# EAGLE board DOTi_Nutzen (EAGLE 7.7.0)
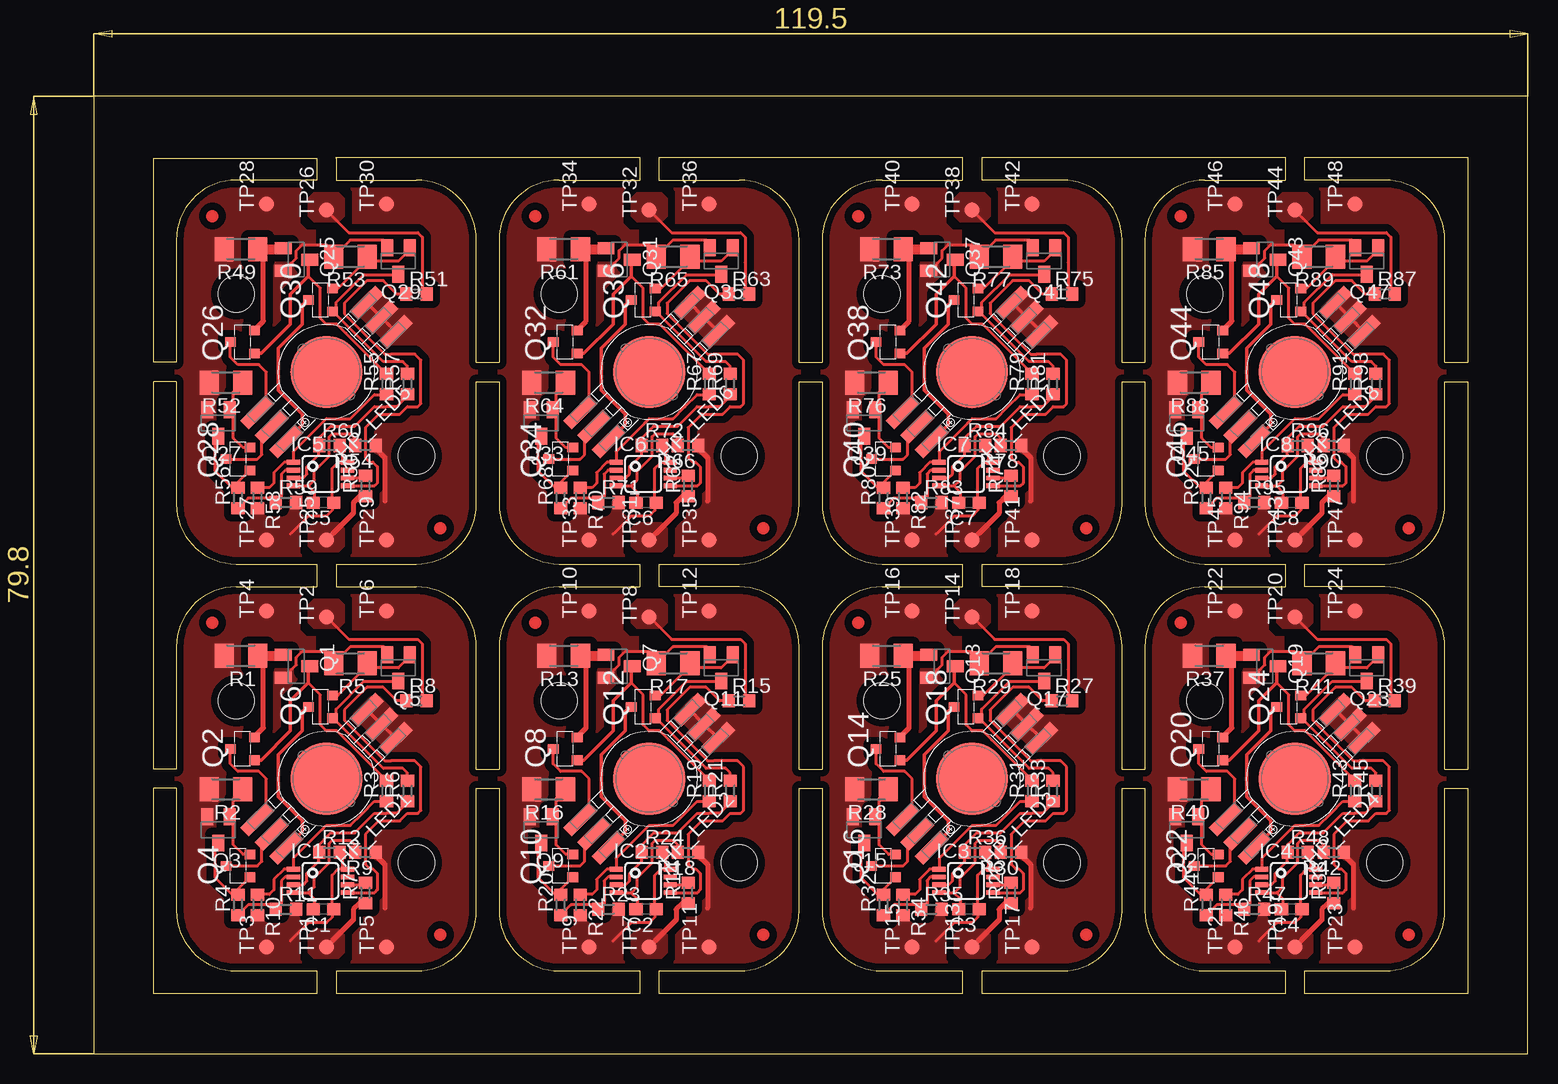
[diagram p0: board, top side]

Size 124.8 x 85.3 mm. Coordinates in mm from the lower left corner, seen from the top.
Outline: 171 segments
Copper layers (1*16): Top 0.035mm / dielectric 1.5mm / Bottom 0.035mm
Design rules "default *": minimum track width 10mil, minimum drill 24mil, track to track 8mil, track to pad 8mil, pad to pad 8mil, via to via 8mil, smd to smd 8mil, copper to edge 20mil, drill to drill 8mil, minimum pad ring 10mil, minimum via ring 8mil, stop-mask expansion 4mil, vias tented up to drill 0mil, thermal gap 10mil
Holes 3 mm at 32.2,15.9 17.2,29.4 59.1,15.9 44.1,29.4 86,15.9 71,29.4 112.9,15.9 97.9,29.4 32.2,49.8 17.2,63.3 59.1,49.8 44.1,63.3 86,49.8 71,63.3 112.9,49.8 97.9,63.3

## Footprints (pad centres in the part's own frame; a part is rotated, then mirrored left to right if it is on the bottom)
C0603 = smd 1.1 x 1: 1 -0.85,0; 2 0.85,0
HP_RGB_LED = smd 3 x 1: 1 -6.45,1.7; 2 -6.45,0; 3 -6.45,-1.7; 4 6.45,-1.7; 5 6.45,0; 6 6.45,1.7 | smd 6 x 6: P$1 0,0
MSOP8 = smd 1.1 x 0.4: 1 -2.25,0.975; 2 -2.25,0.325; 3 -2.25,-0.325; 4 -2.25,-0.975; 5 2.25,-0.975; 6 2.25,-0.325; 7 2.25,0.325; 8 2.25,0.975
SOT23-BEC = smd 1 x 1.4: B -0.95,-1.1; C 0,1.1; E 0.95,-1.1
MICRO3 = smd 0.8 x 0.9: 1 -0.95,-1; 2 0.95,-1; 3 0,1
M1206 = smd 1.6 x 2: 1 -1.4,0; 2 1.4,0
R0603 = smd 1 x 1.1: 1 -0.85,0; 2 0.85,0
B1,27 = smd 1.27 x 1.27: TP 0,0

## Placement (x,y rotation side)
C1  [C0603]  24.45,12.03 180 top
C2  [C0603]  51.35,12.03 180 top
C3  [C0603]  78.25,12.03 180 top
C4  [C0603]  105.15,12.03 180 top
C5  [C0603]  24.45,45.92 180 top
C6  [C0603]  51.35,45.92 180 top
C7  [C0603]  78.25,45.92 180 top
C8  [C0603]  105.15,45.92 180 top
HP_LED1  55-2013  [HP_RGB_LED]  24.7,22.9 225 top
HP_LED2  55-2013  [HP_RGB_LED]  51.6,22.9 225 top
HP_LED3  55-2013  [HP_RGB_LED]  78.5,22.9 225 top
HP_LED4  55-2013  [HP_RGB_LED]  105.4,22.9 225 top
HP_LED5  55-2013  [HP_RGB_LED]  24.7,56.8 225 top
HP_LED6  55-2013  [HP_RGB_LED]  51.6,56.8 225 top
HP_LED7  55-2013  [HP_RGB_LED]  78.5,56.8 225 top
HP_LED8  55-2013  [HP_RGB_LED]  105.4,56.8 225 top
IC1  [MSOP8]  24.2,14.4 0 top
IC2  [MSOP8]  51.1,14.4 0 top
IC3  [MSOP8]  78,14.4 0 top
IC4  [MSOP8]  104.9,14.4 0 top
IC5  [MSOP8]  24.2,48.3 0 top
IC6  [MSOP8]  51.1,48.3 0 top
IC7  [MSOP8]  78,48.3 0 top
IC8  [MSOP8]  104.9,48.3 0 top
Q1  BC857  [SOT23-BEC]  22.2,32.27 270 top
Q2  IRLML5203  [MICRO3]  17.7,25.4 90 top
Q3  BC857  [SOT23-BEC]  15.7,18.65 180 top
Q4  IRLML5203  [MICRO3]  17.32,15.65 90 top
Q5  BC857  [SOT23-BEC]  30.7,32.15 180 top
Q6  IRLML5203  [MICRO3]  24.2,28.9 90 top
Q7  BC857  [SOT23-BEC]  49.1,32.27 270 top
Q8  IRLML5203  [MICRO3]  44.6,25.4 90 top
Q9  BC857  [SOT23-BEC]  42.6,18.65 180 top
Q10  IRLML5203  [MICRO3]  44.22,15.65 90 top
Q11  BC857  [SOT23-BEC]  57.6,32.15 180 top
Q12  IRLML5203  [MICRO3]  51.1,28.9 90 top
Q13  BC857  [SOT23-BEC]  76,32.27 270 top
Q14  IRLML5203  [MICRO3]  71.5,25.4 90 top
Q15  BC857  [SOT23-BEC]  69.5,18.65 180 top
Q16  IRLML5203  [MICRO3]  71.12,15.65 90 top
Q17  BC857  [SOT23-BEC]  84.5,32.15 180 top
Q18  IRLML5203  [MICRO3]  78,28.9 90 top
Q19  BC857  [SOT23-BEC]  102.9,32.27 270 top
Q20  IRLML5203  [MICRO3]  98.4,25.4 90 top
Q21  BC857  [SOT23-BEC]  96.4,18.65 180 top
Q22  IRLML5203  [MICRO3]  98.02,15.65 90 top
Q23  BC857  [SOT23-BEC]  111.4,32.15 180 top
Q24  IRLML5203  [MICRO3]  104.9,28.9 90 top
Q25  BC857  [SOT23-BEC]  22.2,66.17 270 top
Q26  IRLML5203  [MICRO3]  17.7,59.3 90 top
Q27  BC857  [SOT23-BEC]  15.7,52.55 180 top
Q28  IRLML5203  [MICRO3]  17.32,49.55 90 top
Q29  BC857  [SOT23-BEC]  30.7,66.05 180 top
Q30  IRLML5203  [MICRO3]  24.2,62.8 90 top
Q31  BC857  [SOT23-BEC]  49.1,66.17 270 top
Q32  IRLML5203  [MICRO3]  44.6,59.3 90 top
Q33  BC857  [SOT23-BEC]  42.6,52.55 180 top
Q34  IRLML5203  [MICRO3]  44.22,49.55 90 top
Q35  BC857  [SOT23-BEC]  57.6,66.05 180 top
Q36  IRLML5203  [MICRO3]  51.1,62.8 90 top
Q37  BC857  [SOT23-BEC]  76,66.17 270 top
Q38  IRLML5203  [MICRO3]  71.5,59.3 90 top
Q39  BC857  [SOT23-BEC]  69.5,52.55 180 top
Q40  IRLML5203  [MICRO3]  71.12,49.55 90 top
Q41  BC857  [SOT23-BEC]  84.5,66.05 180 top
Q42  IRLML5203  [MICRO3]  78,62.8 90 top
Q43  BC857  [SOT23-BEC]  102.9,66.17 270 top
Q44  IRLML5203  [MICRO3]  98.4,59.3 90 top
Q45  BC857  [SOT23-BEC]  96.4,52.55 180 top
Q46  IRLML5203  [MICRO3]  98.02,49.55 90 top
Q47  BC857  [SOT23-BEC]  111.4,66.05 180 top
Q48  IRLML5203  [MICRO3]  104.9,62.8 90 top
R1  1R8  [M1206]  17.57,33.15 180 top
R2  1R8  [M1206]  16.32,22.02 180 top
R3  4k7  [R0603]  29.7,21.9 90 top
R4  4k7  [R0603]  17.32,12.4 90 top
R5  1R8  [M1206]  26.7,32.52 180 top
R6  4k7  [R0603]  31.45,21.9 90 top
R7  100  [R0603]  27.95,13.4 90 top
R8  100  [R0603]  32.2,29.4 0 top
R9  10  [R0603]  27.95,16.77 180 top
R10  390  [R0603]  18.95,12.4 270 top
R11  390  [R0603]  21.32,12.03 0 top
R12  390  [R0603]  24.95,16.77 0 top
R13  1R8  [M1206]  44.47,33.15 180 top
R14  100  [R0603]  54.85,13.4 90 top
R15  100  [R0603]  59.1,29.4 0 top
R16  1R8  [M1206]  43.22,22.02 180 top
R17  1R8  [M1206]  53.6,32.52 180 top
R18  10  [R0603]  54.85,16.77 180 top
R19  4k7  [R0603]  56.6,21.9 90 top
R20  4k7  [R0603]  44.22,12.4 90 top
R21  4k7  [R0603]  58.35,21.9 90 top
R22  390  [R0603]  45.85,12.4 270 top
R23  390  [R0603]  48.22,12.03 0 top
R24  390  [R0603]  51.85,16.77 0 top
R25  1R8  [M1206]  71.38,33.15 180 top
R26  100  [R0603]  81.75,13.4 90 top
R27  100  [R0603]  86,29.4 0 top
R28  1R8  [M1206]  70.12,22.02 180 top
R29  1R8  [M1206]  80.5,32.52 180 top
R30  10  [R0603]  81.75,16.77 180 top
R31  4k7  [R0603]  83.5,21.9 90 top
R32  4k7  [R0603]  71.12,12.4 90 top
R33  4k7  [R0603]  85.25,21.9 90 top
R34  390  [R0603]  72.75,12.4 270 top
R35  390  [R0603]  75.12,12.03 0 top
R36  390  [R0603]  78.75,16.77 0 top
R37  1R8  [M1206]  98.27,33.15 180 top
R38  100  [R0603]  108.65,13.4 90 top
R39  100  [R0603]  112.9,29.4 0 top
R40  1R8  [M1206]  97.02,22.02 180 top
R41  1R8  [M1206]  107.4,32.52 180 top
R42  10  [R0603]  108.65,16.77 180 top
R43  4k7  [R0603]  110.4,21.9 90 top
R44  4k7  [R0603]  98.02,12.4 90 top
R45  4k7  [R0603]  112.15,21.9 90 top
R46  390  [R0603]  99.65,12.4 270 top
R47  390  [R0603]  102.02,12.03 0 top
R48  390  [R0603]  105.65,16.77 0 top
R49  1R8  [M1206]  17.57,67.05 180 top
R50  100  [R0603]  27.95,47.3 90 top
R51  100  [R0603]  32.2,63.3 0 top
R52  1R8  [M1206]  16.32,55.92 180 top
R53  1R8  [M1206]  26.7,66.42 180 top
R54  10  [R0603]  27.95,50.67 180 top
R55  4k7  [R0603]  29.7,55.8 90 top
R56  4k7  [R0603]  17.32,46.3 90 top
R57  4k7  [R0603]  31.45,55.8 90 top
R58  390  [R0603]  18.95,46.3 270 top
R59  390  [R0603]  21.32,45.92 0 top
R60  390  [R0603]  24.95,50.67 0 top
R61  1R8  [M1206]  44.47,67.05 180 top
R62  100  [R0603]  54.85,47.3 90 top
R63  100  [R0603]  59.1,63.3 0 top
R64  1R8  [M1206]  43.22,55.92 180 top
R65  1R8  [M1206]  53.6,66.42 180 top
R66  10  [R0603]  54.85,50.67 180 top
R67  4k7  [R0603]  56.6,55.8 90 top
R68  4k7  [R0603]  44.22,46.3 90 top
R69  4k7  [R0603]  58.35,55.8 90 top
R70  390  [R0603]  45.85,46.3 270 top
R71  390  [R0603]  48.22,45.92 0 top
R72  390  [R0603]  51.85,50.67 0 top
R73  1R8  [M1206]  71.38,67.05 180 top
R74  100  [R0603]  81.75,47.3 90 top
R75  100  [R0603]  86,63.3 0 top
R76  1R8  [M1206]  70.12,55.92 180 top
R77  1R8  [M1206]  80.5,66.42 180 top
R78  10  [R0603]  81.75,50.67 180 top
R79  4k7  [R0603]  83.5,55.8 90 top
R80  4k7  [R0603]  71.12,46.3 90 top
R81  4k7  [R0603]  85.25,55.8 90 top
R82  390  [R0603]  72.75,46.3 270 top
R83  390  [R0603]  75.12,45.92 0 top
R84  390  [R0603]  78.75,50.67 0 top
R85  1R8  [M1206]  98.27,67.05 180 top
R86  100  [R0603]  108.65,47.3 90 top
R87  100  [R0603]  112.9,63.3 0 top
R88  1R8  [M1206]  97.02,55.92 180 top
R89  1R8  [M1206]  107.4,66.42 180 top
R90  10  [R0603]  108.65,50.67 180 top
R91  4k7  [R0603]  110.4,55.8 90 top
R92  4k7  [R0603]  98.02,46.3 90 top
R93  4k7  [R0603]  112.15,55.8 90 top
R94  390  [R0603]  99.65,46.3 270 top
R95  390  [R0603]  102.02,45.92 0 top
R96  390  [R0603]  105.65,50.67 0 top
TP1  PTR1B1,27  [B1,27]  24.7,8.9 90 top
TP2  PTR1B1,27  [B1,27]  24.7,36.4 90 top
TP3  PTR1B1,27  [B1,27]  19.7,8.9 90 top
TP4  PTR1B1,27  [B1,27]  19.7,36.9 90 top
TP5  PTR1B1,27  [B1,27]  29.7,8.9 90 top
TP6  PTR1B1,27  [B1,27]  29.7,36.9 90 top
TP7  PTR1B1,27  [B1,27]  51.6,8.9 90 top
TP8  PTR1B1,27  [B1,27]  51.6,36.4 90 top
TP9  PTR1B1,27  [B1,27]  46.6,8.9 90 top
TP10  PTR1B1,27  [B1,27]  46.6,36.9 90 top
TP11  PTR1B1,27  [B1,27]  56.6,8.9 90 top
TP12  PTR1B1,27  [B1,27]  56.6,36.9 90 top
TP13  PTR1B1,27  [B1,27]  78.5,8.9 90 top
TP14  PTR1B1,27  [B1,27]  78.5,36.4 90 top
TP15  PTR1B1,27  [B1,27]  73.5,8.9 90 top
TP16  PTR1B1,27  [B1,27]  73.5,36.9 90 top
TP17  PTR1B1,27  [B1,27]  83.5,8.9 90 top
TP18  PTR1B1,27  [B1,27]  83.5,36.9 90 top
TP19  PTR1B1,27  [B1,27]  105.4,8.9 90 top
TP20  PTR1B1,27  [B1,27]  105.4,36.4 90 top
TP21  PTR1B1,27  [B1,27]  100.4,8.9 90 top
TP22  PTR1B1,27  [B1,27]  100.4,36.9 90 top
TP23  PTR1B1,27  [B1,27]  110.4,8.9 90 top
TP24  PTR1B1,27  [B1,27]  110.4,36.9 90 top
TP25  PTR1B1,27  [B1,27]  24.7,42.8 90 top
TP26  PTR1B1,27  [B1,27]  24.7,70.3 90 top
TP27  PTR1B1,27  [B1,27]  19.7,42.8 90 top
TP28  PTR1B1,27  [B1,27]  19.7,70.8 90 top
TP29  PTR1B1,27  [B1,27]  29.7,42.8 90 top
TP30  PTR1B1,27  [B1,27]  29.7,70.8 90 top
TP31  PTR1B1,27  [B1,27]  51.6,42.8 90 top
TP32  PTR1B1,27  [B1,27]  51.6,70.3 90 top
TP33  PTR1B1,27  [B1,27]  46.6,42.8 90 top
TP34  PTR1B1,27  [B1,27]  46.6,70.8 90 top
TP35  PTR1B1,27  [B1,27]  56.6,42.8 90 top
TP36  PTR1B1,27  [B1,27]  56.6,70.8 90 top
TP37  PTR1B1,27  [B1,27]  78.5,42.8 90 top
TP38  PTR1B1,27  [B1,27]  78.5,70.3 90 top
TP39  PTR1B1,27  [B1,27]  73.5,42.8 90 top
TP40  PTR1B1,27  [B1,27]  73.5,70.8 90 top
TP41  PTR1B1,27  [B1,27]  83.5,42.8 90 top
TP42  PTR1B1,27  [B1,27]  83.5,70.8 90 top
TP43  PTR1B1,27  [B1,27]  105.4,42.8 90 top
TP44  PTR1B1,27  [B1,27]  105.4,70.3 90 top
TP45  PTR1B1,27  [B1,27]  100.4,42.8 90 top
TP46  PTR1B1,27  [B1,27]  100.4,70.8 90 top
TP47  PTR1B1,27  [B1,27]  110.4,42.8 90 top
TP48  PTR1B1,27  [B1,27]  110.4,70.8 90 top

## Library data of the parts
C1-C8 R1-R96 = rcl
HP_LED1-HP_LED8 = RGB_HP_LED
IC1-IC8 = WS2812
Q1 Q3 Q5 Q7 Q9 Q11 Q13 Q15 Q17 Q19 Q21 Q23 Q25 Q27 Q29 Q31 Q33 Q35 Q37 Q39 Q41 Q43 Q45 Q47 = transistor-pnp
Q2 Q4 Q6 Q8 Q10 Q12 Q14 Q16 Q18 Q20 Q22 Q24 Q26 Q28 Q30 Q32 Q34 Q36 Q38 Q40 Q42 Q44 Q46 Q48 = transistor-power
TP1-TP48 = testpad

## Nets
B: IC1.3 R6.1 R12.1
B1: IC2.3 R21.1 R24.1
B2: IC3.3 R33.1 R36.1
B3: IC4.3 R45.1 R48.1
B4: IC5.3 R57.1 R60.1
B5: IC6.3 R69.1 R72.1
B6: IC7.3 R81.1 R84.1
B7: IC8.3 R93.1 R96.1
DI: IC1.6 R7.2
DI1: IC2.6 R14.2
DI2: IC3.6 R26.2
DI3: IC4.6 R38.2
DI4: IC5.6 R50.2
DI5: IC6.6 R62.2
DI6: IC7.6 R74.2
DI7: IC8.6 R86.2
DIN: R7.1 TP1.TP
DIN1: R14.1 TP7.TP
DIN2: R26.1 TP13.TP
DIN3: R38.1 TP19.TP
DIN4: R50.1 TP25.TP
DIN5: R62.1 TP31.TP
DIN6: R74.1 TP37.TP
DIN7: R86.1 TP43.TP
DO: IC1.5 R8.1
DO1: IC2.5 R15.1
DO2: IC3.5 R27.1
DO3: IC4.5 R39.1
DO4: IC5.5 R51.1
DO5: IC6.5 R63.1
DO6: IC7.5 R75.1
DO7: IC8.5 R87.1
DOUT: R8.2 TP2.TP
DOUT1: R15.2 TP8.TP
DOUT2: R27.2 TP14.TP
DOUT3: R39.2 TP20.TP
DOUT4: R51.2 TP26.TP
DOUT5: R63.2 TP32.TP
DOUT6: R75.2 TP38.TP
DOUT7: R87.2 TP44.TP
G: IC1.2 R4.1 R11.1
G1: IC2.2 R20.1 R23.1
G2: IC3.2 R32.1 R35.1
G3: IC4.2 R44.1 R47.1
G4: IC5.2 R56.1 R59.1
G5: IC6.2 R68.1 R71.1
G6: IC7.2 R80.1 R83.1
G7: IC8.2 R92.1 R95.1
GND: HP_LED1.1 HP_LED1.2 HP_LED1.3 R9.1 TP5.TP TP6.TP
GND1: HP_LED2.1 HP_LED2.2 HP_LED2.3 R18.1 TP11.TP TP12.TP
GND2: HP_LED3.1 HP_LED3.2 HP_LED3.3 R30.1 TP17.TP TP18.TP
GND3: HP_LED4.1 HP_LED4.2 HP_LED4.3 R42.1 TP23.TP TP24.TP
GND8: HP_LED5.1 HP_LED5.2 HP_LED5.3 R54.1 TP29.TP TP30.TP
GND9: HP_LED6.1 HP_LED6.2 HP_LED6.3 R66.1 TP35.TP TP36.TP
GND10: HP_LED7.1 HP_LED7.2 HP_LED7.3 R78.1 TP41.TP TP42.TP
GND11: HP_LED8.1 HP_LED8.2 HP_LED8.3 R90.1 TP47.TP TP48.TP
N$1: HP_LED1.5 Q4.3
N$2: Q1.B Q2.2 R1.1
N$3: Q1.C Q2.1 R3.2
N$4: HP_LED1.4 Q2.3
N$5: HP_LED1.6 Q6.3
N$6: Q3.B Q4.2 R2.1
N$7: Q5.B Q6.2 R5.1
N$8: Q7.B Q8.2 R13.1
N$9: Q3.C Q4.1 R4.2
N$10: HP_LED2.4 Q8.3
N$11: Q5.C Q6.1 R6.2
N$12: C1.2 IC1.4 R9.2
N$13: HP_LED2.5 Q10.3
N$14: HP_LED2.6 Q12.3
N$15: Q7.C Q8.1 R19.2
N$16: Q9.B Q10.2 R16.1
N$17: Q9.C Q10.1 R20.2
N$18: Q11.B Q12.2 R17.1
N$19: Q11.C Q12.1 R21.2
N$20: C2.2 IC2.4 R18.2
N$21: Q13.B Q14.2 R25.1
N$22: HP_LED3.4 Q14.3
N$23: HP_LED3.5 Q16.3
N$24: HP_LED3.6 Q18.3
N$25: Q13.C Q14.1 R31.2
N$26: Q15.B Q16.2 R28.1
N$27: Q15.C Q16.1 R32.2
N$28: Q17.B Q18.2 R29.1
N$29: Q17.C Q18.1 R33.2
N$30: C3.2 IC3.4 R30.2
N$31: Q19.B Q20.2 R37.1
N$32: HP_LED4.4 Q20.3
N$33: HP_LED4.5 Q22.3
N$34: HP_LED4.6 Q24.3
N$35: Q19.C Q20.1 R43.2
N$36: Q21.B Q22.2 R40.1
N$37: Q21.C Q22.1 R44.2
N$38: Q23.B Q24.2 R41.1
N$39: Q23.C Q24.1 R45.2
N$40: C4.2 IC4.4 R42.2
N$41: Q25.B Q26.2 R49.1
N$42: HP_LED5.4 Q26.3
N$43: HP_LED5.5 Q28.3
N$44: HP_LED5.6 Q30.3
N$45: Q25.C Q26.1 R55.2
N$46: Q27.B Q28.2 R52.1
N$47: Q27.C Q28.1 R56.2
N$48: Q29.B Q30.2 R53.1
N$49: Q29.C Q30.1 R57.2
N$50: C5.2 IC5.4 R54.2
N$51: Q31.B Q32.2 R61.1
N$52: HP_LED6.4 Q32.3
N$53: HP_LED6.5 Q34.3
N$54: HP_LED6.6 Q36.3
N$55: Q31.C Q32.1 R67.2
N$56: Q33.B Q34.2 R64.1
N$57: Q33.C Q34.1 R68.2
N$58: Q35.B Q36.2 R65.1
N$59: Q35.C Q36.1 R69.2
N$60: C6.2 IC6.4 R66.2
N$61: Q37.B Q38.2 R73.1
N$62: HP_LED7.4 Q38.3
N$63: HP_LED7.5 Q40.3
N$64: HP_LED7.6 Q42.3
N$65: Q37.C Q38.1 R79.2
N$66: Q39.B Q40.2 R76.1
N$67: Q39.C Q40.1 R80.2
N$68: Q41.B Q42.2 R77.1
N$69: Q41.C Q42.1 R81.2
N$70: C7.2 IC7.4 R78.2
N$71: Q43.B Q44.2 R85.1
N$72: HP_LED8.4 Q44.3
N$73: HP_LED8.5 Q46.3
N$74: HP_LED8.6 Q48.3
N$75: Q43.C Q44.1 R91.2
N$76: Q45.B Q46.2 R88.1
N$77: Q45.C Q46.1 R92.2
N$78: Q47.B Q48.2 R89.1
N$79: Q47.C Q48.1 R93.2
N$80: C8.2 IC8.4 R90.2
R: IC1.1 R3.1 R10.1
R1: IC2.1 R19.1 R22.1
R2: IC3.1 R31.1 R34.1
R3: IC4.1 R43.1 R46.1
R4: IC5.1 R55.1 R58.1
R5: IC6.1 R67.1 R70.1
R6: IC7.1 R79.1 R82.1
R7: IC8.1 R91.1 R94.1
VCC: C1.1 IC1.8 Q1.E Q3.E Q5.E R1.2 R2.2 R5.2 R10.2 R11.2 R12.2 TP3.TP TP4.TP
VCC1: C2.1 IC2.8 Q7.E Q9.E Q11.E R13.2 R16.2 R17.2 R22.2 R23.2 R24.2 TP9.TP TP10.TP
VCC2: C3.1 IC3.8 Q13.E Q15.E Q17.E R25.2 R28.2 R29.2 R34.2 R35.2 R36.2 TP15.TP TP16.TP
VCC3: C4.1 IC4.8 Q19.E Q21.E Q23.E R37.2 R40.2 R41.2 R46.2 R47.2 R48.2 TP21.TP TP22.TP
VCC8: C5.1 IC5.8 Q25.E Q27.E Q29.E R49.2 R52.2 R53.2 R58.2 R59.2 R60.2 TP27.TP TP28.TP
VCC9: C6.1 IC6.8 Q31.E Q33.E Q35.E R61.2 R64.2 R65.2 R70.2 R71.2 R72.2 TP33.TP TP34.TP
VCC10: C7.1 IC7.8 Q37.E Q39.E Q41.E R73.2 R76.2 R77.2 R82.2 R83.2 R84.2 TP39.TP TP40.TP
VCC11: C8.1 IC8.8 Q43.E Q45.E Q47.E R85.2 R88.2 R89.2 R94.2 R95.2 R96.2 TP45.TP TP46.TP

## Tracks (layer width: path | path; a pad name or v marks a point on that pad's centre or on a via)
B
  Top 0.254: IC1.3 22.75,14.07 23.07,14.4 23.07,15.03 24.07,16.02 24.07,16.75 R12.1 24.1,17.43 24.82,18.15 25.07,18.4 27.07,18.4 28.7,20.02 29.7,20.02 30.57,20.02 31.45,20.9
  Top 0.305: R6.1 31.45,20.9
B1
  Top 0.254: IC2.3 49.65,14.07 49.97,14.4 49.97,15.03 50.97,16.02 50.97,16.75 R24.1 51,17.43 51.72,18.15 51.97,18.4 53.97,18.4 55.6,20.02 56.6,20.02 57.47,20.02 58.35,20.9
  Top 0.305: R21.1 58.35,20.9
B2
  Top 0.254: IC3.3 76.55,14.07 76.88,14.4 76.88,15.03 77.88,16.02 77.88,16.75 R36.1 77.9,17.43 78.62,18.15 78.88,18.4 80.88,18.4 82.5,20.02 83.5,20.02 84.38,20.02 85.25,20.9
  Top 0.305: R33.1 85.25,20.9
B3
  Top 0.254: IC4.3 103.45,14.07 103.77,14.4 103.77,15.03 104.77,16.02 104.77,16.75 R48.1 104.8,17.43 105.52,18.15 105.77,18.4 107.77,18.4 109.4,20.02 110.4,20.02 111.27,20.02 112.15,20.9
  Top 0.305: R45.1 112.15,20.9
B4
  Top 0.254: IC5.3 22.75,47.98 23.07,48.3 23.07,48.92 24.07,49.92 24.07,50.65 R60.1 24.1,51.33 24.82,52.05 25.07,52.3 27.07,52.3 28.7,53.92 29.7,53.92 30.57,53.92 31.45,54.8
  Top 0.305: R57.1 31.45,54.8
B5
  Top 0.254: IC6.3 49.65,47.98 49.97,48.3 49.97,48.92 50.97,49.92 50.97,50.65 R72.1 51,51.33 51.72,52.05 51.97,52.3 53.97,52.3 55.6,53.92 56.6,53.92 57.47,53.92 58.35,54.8
  Top 0.305: R69.1 58.35,54.8
B6
  Top 0.254: IC7.3 76.55,47.98 76.88,48.3 76.88,48.92 77.88,49.92 77.88,50.65 R84.1 77.9,51.33 78.62,52.05 78.88,52.3 80.88,52.3 82.5,53.92 83.5,53.92 84.38,53.92 85.25,54.8
  Top 0.305: R81.1 85.25,54.8
B7
  Top 0.254: IC8.3 103.45,47.98 103.77,48.3 103.77,48.92 104.77,49.92 104.77,50.65 R96.1 104.8,51.33 105.52,52.05 105.77,52.3 107.77,52.3 109.4,53.92 110.4,53.92 111.27,53.92 112.15,54.8
  Top 0.305: R93.1 112.15,54.8
DI
  Top 0.254: IC1.6 27.9,14.07 R7.2
DI1
  Top 0.254: IC2.6 54.8,14.07 R14.2
DI2
  Top 0.254: IC3.6 81.7,14.07 R26.2
DI3
  Top 0.254: IC4.6 108.6,14.07 R38.2
DI4
  Top 0.254: IC5.6 27.9,47.98 R50.2
DI5
  Top 0.254: IC6.6 54.8,47.98 R62.2
DI6
  Top 0.254: IC7.6 81.7,47.98 R74.2
DI7
  Top 0.254: IC8.6 108.6,47.98 R86.2
DIN
  Top 0.254: 25.2,9.4 TP1.TP
  Top 0.406: R7.1 27.48,12.55 26.95,12.03 26.95,11.15 26.32,10.53 25.2,9.4
  pour Top (no thermals): 25.7,7.9 23.7,7.9 23.2,8.4 23.2,9.9 23.7,10.4 25.7,10.4 26.2,9.9 26.2,8.4
DIN1
  Top 0.254: 52.1,9.4 TP7.TP
  Top 0.406: R14.1 54.38,12.55 53.85,12.03 53.85,11.15 53.22,10.53 52.1,9.4
  pour Top (no thermals): 52.6,7.9 50.6,7.9 50.1,8.4 50.1,9.9 50.6,10.4 52.6,10.4 53.1,9.9 53.1,8.4
DIN2
  Top 0.254: 79,9.4 TP13.TP
  Top 0.406: R26.1 81.27,12.55 80.75,12.03 80.75,11.15 80.12,10.53 79,9.4
  pour Top (no thermals): 79.5,7.9 77.5,7.9 77,8.4 77,9.9 77.5,10.4 79.5,10.4 80,9.9 80,8.4
DIN3
  Top 0.254: 105.9,9.4 TP19.TP
  Top 0.406: R38.1 108.17,12.55 107.65,12.03 107.65,11.15 107.02,10.53 105.9,9.4
  pour Top (no thermals): 106.4,7.9 104.4,7.9 103.9,8.4 103.9,9.9 104.4,10.4 106.4,10.4 106.9,9.9 106.9,8.4
DIN4
  Top 0.254: 25.2,43.3 TP25.TP
  Top 0.406: R50.1 27.48,46.45 26.95,45.92 26.95,45.05 26.32,44.42 25.2,43.3
  pour Top (no thermals): 25.7,41.8 23.7,41.8 23.2,42.3 23.2,43.8 23.7,44.3 25.7,44.3 26.2,43.8 26.2,42.3
DIN5
  Top 0.254: 52.1,43.3 TP31.TP
  Top 0.406: R62.1 54.38,46.45 53.85,45.92 53.85,45.05 53.22,44.42 52.1,43.3
  pour Top (no thermals): 52.6,41.8 50.6,41.8 50.1,42.3 50.1,43.8 50.6,44.3 52.6,44.3 53.1,43.8 53.1,42.3
DIN6
  Top 0.254: 79,43.3 TP37.TP
  Top 0.406: R74.1 81.27,46.45 80.75,45.92 80.75,45.05 80.12,44.42 79,43.3
  pour Top (no thermals): 79.5,41.8 77.5,41.8 77,42.3 77,43.8 77.5,44.3 79.5,44.3 80,43.8 80,42.3
DIN7
  Top 0.254: 105.9,43.3 TP43.TP
  Top 0.406: R86.1 108.17,46.45 107.65,45.92 107.65,45.05 107.02,44.42 105.9,43.3
  pour Top (no thermals): 106.4,41.8 104.4,41.8 103.9,42.3 103.9,43.8 104.4,44.3 106.4,44.3 106.9,43.8 106.9,42.3
DO
  Top 0.254: R8.1 30.57,29.4 29.45,30.52 28.07,30.52 27.7,30.15 26.2,28.65 26.2,27.77 29.57,24.4 30.07,24.4 32.07,24.4 32.57,23.9 32.57,20.27 32.32,20.02 31.45,20.02 30.82,19.4 29.07,19.4 28.32,18.65 27.95,18.27 27.95,15.78 28.32,15.4 28.57,15.4 28.95,15.03 28.95,13.65 28.73,13.43 IC1.5
DO1
  Top 0.254: R15.1 57.47,29.4 56.35,30.52 54.97,30.52 54.6,30.15 53.1,28.65 53.1,27.77 56.47,24.4 56.97,24.4 58.97,24.4 59.47,23.9 59.47,20.27 59.22,20.02 58.35,20.02 57.72,19.4 55.97,19.4 55.22,18.65 54.85,18.27 54.85,15.78 55.22,15.4 55.47,15.4 55.85,15.03 55.85,13.65 55.62,13.43 IC2.5
DO2
  Top 0.254: R27.1 84.38,29.4 83.25,30.52 81.88,30.52 81.5,30.15 80,28.65 80,27.77 83.38,24.4 83.88,24.4 85.88,24.4 86.38,23.9 86.38,20.27 86.12,20.02 85.25,20.02 84.62,19.4 82.88,19.4 82.12,18.65 81.75,18.27 81.75,15.78 82.12,15.4 82.38,15.4 82.75,15.03 82.75,13.65 82.52,13.43 IC3.5
DO3
  Top 0.254: R39.1 111.27,29.4 110.15,30.52 108.77,30.52 108.4,30.15 106.9,28.65 106.9,27.77 110.27,24.4 110.77,24.4 112.77,24.4 113.27,23.9 113.27,20.27 113.02,20.02 112.15,20.02 111.52,19.4 109.77,19.4 109.02,18.65 108.65,18.27 108.65,15.78 109.02,15.4 109.27,15.4 109.65,15.03 109.65,13.65 109.42,13.43 IC4.5
DO4
  Top 0.254: R51.1 30.57,63.3 29.45,64.42 28.07,64.42 27.7,64.05 26.2,62.55 26.2,61.67 29.57,58.3 30.07,58.3 32.07,58.3 32.57,57.8 32.57,54.17 32.32,53.92 31.45,53.92 30.82,53.3 29.07,53.3 28.32,52.55 27.95,52.17 27.95,49.67 28.32,49.3 28.57,49.3 28.95,48.92 28.95,47.55 28.73,47.33 IC5.5
DO5
  Top 0.254: R63.1 57.47,63.3 56.35,64.42 54.97,64.42 54.6,64.05 53.1,62.55 53.1,61.67 56.47,58.3 56.97,58.3 58.97,58.3 59.47,57.8 59.47,54.17 59.22,53.92 58.35,53.92 57.72,53.3 55.97,53.3 55.22,52.55 54.85,52.17 54.85,49.67 55.22,49.3 55.47,49.3 55.85,48.92 55.85,47.55 55.62,47.33 IC6.5
DO6
  Top 0.254: R75.1 84.38,63.3 83.25,64.42 81.88,64.42 81.5,64.05 80,62.55 80,61.67 83.38,58.3 83.88,58.3 85.88,58.3 86.38,57.8 86.38,54.17 86.12,53.92 85.25,53.92 84.62,53.3 82.88,53.3 82.12,52.55 81.75,52.17 81.75,49.67 82.12,49.3 82.38,49.3 82.75,48.92 82.75,47.55 82.52,47.33 IC7.5
DO7
  Top 0.254: R87.1 111.27,63.3 110.15,64.42 108.77,64.42 108.4,64.05 106.9,62.55 106.9,61.67 110.27,58.3 110.77,58.3 112.77,58.3 113.27,57.8 113.27,54.17 113.02,53.92 112.15,53.92 111.52,53.3 109.77,53.3 109.02,52.55 108.65,52.17 108.65,49.67 109.02,49.3 109.27,49.3 109.65,48.92 109.65,47.55 109.42,47.33 IC8.5
DOUT
  Top 0.254: TP2.TP 26.57,34.52 32.32,34.52 32.7,34.15 32.7,32.02 32.7,29.9 33.2,29.43 R8.2
  pour Top (isolate 0.406, no thermals): 23.7,35.4 23.2,35.9 23.2,37.4 23.7,37.9 25.7,37.9 26.2,37.4 26.2,35.9 25.7,35.4
DOUT1
  Top 0.254: TP8.TP 53.47,34.52 59.22,34.52 59.6,34.15 59.6,32.02 59.6,29.9 60.1,29.43 R15.2
  pour Top (isolate 0.406, no thermals): 50.6,35.4 50.1,35.9 50.1,37.4 50.6,37.9 52.6,37.9 53.1,37.4 53.1,35.9 52.6,35.4
DOUT2
  Top 0.254: TP14.TP 80.38,34.52 86.12,34.52 86.5,34.15 86.5,32.02 86.5,29.9 87,29.43 R27.2
  pour Top (isolate 0.406, no thermals): 77.5,35.4 77,35.9 77,37.4 77.5,37.9 79.5,37.9 80,37.4 80,35.9 79.5,35.4
DOUT3
  Top 0.254: TP20.TP 107.27,34.52 113.02,34.52 113.4,34.15 113.4,32.02 113.4,29.9 113.9,29.43 R39.2
  pour Top (isolate 0.406, no thermals): 104.4,35.4 103.9,35.9 103.9,37.4 104.4,37.9 106.4,37.9 106.9,37.4 106.9,35.9 106.4,35.4
DOUT4
  Top 0.254: TP26.TP 26.57,68.42 32.32,68.42 32.7,68.05 32.7,65.92 32.7,63.8 33.2,63.33 R51.2
  pour Top (isolate 0.406, no thermals): 23.7,69.3 23.2,69.8 23.2,71.3 23.7,71.8 25.7,71.8 26.2,71.3 26.2,69.8 25.7,69.3
DOUT5
  Top 0.254: TP32.TP 53.47,68.42 59.22,68.42 59.6,68.05 59.6,65.92 59.6,63.8 60.1,63.33 R63.2
  pour Top (isolate 0.406, no thermals): 50.6,69.3 50.1,69.8 50.1,71.3 50.6,71.8 52.6,71.8 53.1,71.3 53.1,69.8 52.6,69.3
DOUT6
  Top 0.254: TP38.TP 80.38,68.42 86.12,68.42 86.5,68.05 86.5,65.92 86.5,63.8 87,63.33 R75.2
  pour Top (isolate 0.406, no thermals): 77.5,69.3 77,69.8 77,71.3 77.5,71.8 79.5,71.8 80,71.3 80,69.8 79.5,69.3
DOUT7
  Top 0.254: TP44.TP 107.27,68.42 113.02,68.42 113.4,68.05 113.4,65.92 113.4,63.8 113.9,63.33 R87.2
  pour Top (isolate 0.406, no thermals): 104.4,69.3 103.9,69.8 103.9,71.3 104.4,71.8 106.4,71.8 106.9,71.3 106.9,69.8 106.4,69.3
G
  Top 0.254: IC1.2 21.27,14.72 20.95,14.4 20.95,12.5 R11.1 20.48,12.12 20.2,12.4 18.18,12.4 R4.1
G1
  Top 0.254: IC2.2 48.17,14.72 47.85,14.4 47.85,12.5 R23.1 47.38,12.12 47.1,12.4 45.07,12.4 R20.1
G2
  Top 0.254: IC3.2 75.08,14.72 74.75,14.4 74.75,12.5 R35.1 74.27,12.12 74,12.4 71.97,12.4 R32.1
G3
  Top 0.254: IC4.2 101.97,14.72 101.65,14.4 101.65,12.5 R47.1 101.17,12.12 100.9,12.4 98.88,12.4 R44.1
G4
  Top 0.254: IC5.2 21.27,48.62 20.95,48.3 20.95,46.4 R59.1 20.48,46.02 20.2,46.3 18.18,46.3 R56.1
G5
  Top 0.254: IC6.2 48.17,48.62 47.85,48.3 47.85,46.4 R71.1 47.38,46.02 47.1,46.3 45.07,46.3 R68.1
G6
  Top 0.254: IC7.2 75.08,48.62 74.75,48.3 74.75,46.4 R83.1 74.27,46.02 74,46.3 71.97,46.3 R80.1
G7
  Top 0.254: IC8.2 101.97,48.62 101.65,48.3 101.65,46.4 R95.1 101.17,46.02 100.9,46.3 98.88,46.3 R92.1
GND
  Top 0.305: HP_LED1.3 HP_LED1.2 HP_LED1.1 | R9.1 28.8,16.55
  Top 0.406: 28.8,16.55 29.57,15.78 29.57,12.15
  pour Top (isolate 0.61, rank 2, no thermals): 25.7,6.9 25.7,38.9 37.2,38.9 37.2,6.9
GND1
  Top 0.305: HP_LED2.3 HP_LED2.2 HP_LED2.1 | R18.1 55.7,16.55
  Top 0.406: 55.7,16.55 56.47,15.78 56.47,12.15
  pour Top (isolate 0.61, rank 2, no thermals): 52.6,6.9 52.6,38.9 64.1,38.9 64.1,6.9
GND2
  Top 0.305: HP_LED3.3 HP_LED3.2 HP_LED3.1 | R30.1 82.6,16.55
  Top 0.406: 82.6,16.55 83.38,15.78 83.38,12.15
  pour Top (isolate 0.61, rank 2, no thermals): 79.5,6.9 79.5,38.9 91,38.9 91,6.9
GND3
  Top 0.305: HP_LED4.3 HP_LED4.2 HP_LED4.1 | R42.1 109.5,16.55
  Top 0.406: 109.5,16.55 110.27,15.78 110.27,12.15
  pour Top (isolate 0.61, rank 2, no thermals): 106.4,6.9 106.4,38.9 117.9,38.9 117.9,6.9
GND8
  Top 0.305: HP_LED5.3 HP_LED5.2 HP_LED5.1 | R54.1 28.8,50.45
  Top 0.406: 28.8,50.45 29.57,49.67 29.57,46.05
  pour Top (isolate 0.61, rank 2, no thermals): 25.7,40.8 25.7,72.8 37.2,72.8 37.2,40.8
GND9
  Top 0.305: HP_LED6.3 HP_LED6.2 HP_LED6.1 | R66.1 55.7,50.45
  Top 0.406: 55.7,50.45 56.47,49.67 56.47,46.05
  pour Top (isolate 0.61, rank 2, no thermals): 52.6,40.8 52.6,72.8 64.1,72.8 64.1,40.8
GND10
  Top 0.305: HP_LED7.3 HP_LED7.2 HP_LED7.1 | R78.1 82.6,50.45
  Top 0.406: 82.6,50.45 83.38,49.67 83.38,46.05
  pour Top (isolate 0.61, rank 2, no thermals): 79.5,40.8 79.5,72.8 91,72.8 91,40.8
GND11
  Top 0.305: HP_LED8.3 HP_LED8.2 HP_LED8.1 | R90.1 109.5,50.45
  Top 0.406: 109.5,50.45 110.27,49.67 110.27,46.05
  pour Top (isolate 0.61, rank 2, no thermals): 106.4,40.8 106.4,72.8 117.9,72.8 117.9,40.8
N$1
  Top 0.254: Q4.3 18.95,15.65 19.32,16.02 19.32,17.52 HP_LED1.5
N$2
  Top 0.305: 20.77,33.15 Q1.B | Q2.2 18.7,26.4
  Top 0.406: 18.7,26.4 19.45,27.15 19.45,32.55 R1.1
  Top 0.813: R1.1 20.77,33.15
N$3  (1 unrouted)
  Top 0.254: 23.2,30.9 24.2,29.9 24.2,27.4 24.7,26.9 25.57,26.9 26.32,26.15 29.7,22.77 30.07,22.77
  Top 0.305: 19.15,24.45 Q2.1 19.25,24.45 21.7,26.9 21.7,29.4 23.2,30.9 23.2,32.17 Q1.C
N$4
  Top 0.254: HP_LED1.4 18.94,19.64 19.7,20.4 19.7,22.9 19.07,23.52 17.32,23.52 16.7,24.15 Q2.3
N$5
  Top 0.305: HP_LED1.6 22.7,18.5 22.7,18.9 22.7,19.4 20.7,21.4 20.7,23.4 20.7,24.9 22.7,26.9 22.7,28.52 Q6.3
N$6
  Top 0.254: Q4.2 17.75,16.6 16.95,17.4 16.95,19.45 Q3.B 16.65,19.85 16.95,20.15 16.95,21.25 R2.1
N$7
  Top 0.254: Q6.2 25.65,29.85 28.07,32.27 | 28.07,32.27 28.07,32.88 R5.1 | Q5.B 31.65,33.1 30.7,32.15 28.2,32.15 28.07,32.27
N$8
  Top 0.305: 47.67,33.15 Q7.B | Q8.2 45.6,26.4
  Top 0.406: 45.6,26.4 46.35,27.15 46.35,32.55 R13.1
  Top 0.813: R13.1 47.67,33.15
N$9
  Top 0.254: Q4.1 17.32,13.7 R4.2 16.85,13.25 15.45,14.65 15.45,17.3 Q3.C 15.7,17.52 15.45,17.15
N$10
  Top 0.254: HP_LED2.4 45.84,19.64 46.6,20.4 46.6,22.9 45.97,23.52 44.22,23.52 43.6,24.15 Q8.3
N$11
  Top 0.254: Q6.1 25.2,27.9 25.45,27.77 29.45,23.77 31.07,23.77 31.45,23.4 R6.2 | 25.5,27.95 25.5,28.7 27.82,31.02 30.68,31.02 Q5.C
  Top 0.305: Q6.1 25.5,27.95
N$12
  Top 0.254: IC1.4 23.18,13.43 | 23.18,13.43 23.7,12.9 23.7,12.12 C1.2 | 23.18,13.43 23.23,13.43 23.7,13.9 23.7,14.65 24.95,15.9 24.95,17.52 25.2,17.77 26.7,17.77 27.07,17.4 27.07,16.8 R9.2
  Top 0.305: C1.2 23.6,12.25 23.57,12.28 23.57,12.03 C1.2 | C1.2 23.7,12.03
N$13
  Top 0.254: Q10.3 45.85,15.65 46.22,16.02 46.22,17.52 HP_LED2.5
N$14
  Top 0.305: HP_LED2.6 49.6,18.5 49.6,18.9 49.6,19.4 47.6,21.4 47.6,23.4 47.6,24.9 49.6,26.9 49.6,28.52 Q12.3
N$15  (1 unrouted)
  Top 0.254: 50.1,30.9 51.1,29.9 51.1,27.4 51.6,26.9 52.47,26.9 53.22,26.15 56.6,22.77 56.97,22.77
  Top 0.305: 46.05,24.45 Q8.1 46.15,24.45 48.6,26.9 48.6,29.4 50.1,30.9 50.1,32.17 Q7.C
N$16
  Top 0.254: Q10.2 44.65,16.6 43.85,17.4 43.85,19.45 Q9.B 43.55,19.85 43.85,20.15 43.85,21.25 R16.1
N$17
  Top 0.254: Q10.1 44.22,13.7 R20.2 43.75,13.25 42.35,14.65 42.35,17.3 Q9.C 42.6,17.52 42.35,17.15
N$18
  Top 0.254: Q12.2 52.55,29.85 54.97,32.27 | 54.97,32.27 54.97,32.88 R17.1 | Q11.B 58.55,33.1 57.6,32.15 55.1,32.15 54.97,32.27
N$19
  Top 0.254: Q12.1 52.1,27.9 52.35,27.77 56.35,23.77 57.97,23.77 58.35,23.4 R21.2 | 52.4,27.95 52.4,28.7 54.72,31.02 57.57,31.02 Q11.C
  Top 0.305: Q12.1 52.4,27.95
N$20
  Top 0.254: IC2.4 50.07,13.43 | 50.07,13.43 50.6,12.9 50.6,12.12 C2.2 | 50.07,13.43 50.12,13.43 50.6,13.9 50.6,14.65 51.85,15.9 51.85,17.52 52.1,17.77 53.6,17.77 53.97,17.4 53.97,16.8 R18.2
  Top 0.305: C2.2 50.5,12.25 50.47,12.28 50.47,12.03 C2.2 | C2.2 50.6,12.03
N$21
  Top 0.305: 74.58,33.15 Q13.B | Q14.2 72.5,26.4
  Top 0.406: 72.5,26.4 73.25,27.15 73.25,32.55 R25.1
  Top 0.813: R25.1 74.58,33.15
N$22
  Top 0.254: HP_LED3.4 72.74,19.64 73.5,20.4 73.5,22.9 72.88,23.52 71.12,23.52 70.5,24.15 Q14.3
N$23
  Top 0.254: Q16.3 72.75,15.65 73.12,16.02 73.12,17.52 HP_LED3.5
N$24
  Top 0.305: HP_LED3.6 76.5,18.5 76.5,18.9 76.5,19.4 74.5,21.4 74.5,23.4 74.5,24.9 76.5,26.9 76.5,28.52 Q18.3
N$25  (1 unrouted)
  Top 0.254: 77,30.9 78,29.9 78,27.4 78.5,26.9 79.38,26.9 80.12,26.15 83.5,22.77 83.88,22.77
  Top 0.305: 72.95,24.45 Q14.1 73.05,24.45 75.5,26.9 75.5,29.4 77,30.9 77,32.17 Q13.C
N$26
  Top 0.254: Q16.2 71.55,16.6 70.75,17.4 70.75,19.45 Q15.B 70.45,19.85 70.75,20.15 70.75,21.25 R28.1
N$27
  Top 0.254: Q16.1 71.12,13.7 R32.2 70.65,13.25 69.25,14.65 69.25,17.3 Q15.C 69.5,17.52 69.25,17.15
N$28
  Top 0.254: Q18.2 79.45,29.85 81.88,32.27 | 81.88,32.27 81.88,32.88 R29.1 | Q17.B 85.45,33.1 84.5,32.15 82,32.15 81.88,32.27
N$29
  Top 0.254: Q18.1 79,27.9 79.25,27.77 83.25,23.77 84.88,23.77 85.25,23.4 R33.2 | 79.3,27.95 79.3,28.7 81.62,31.02 84.47,31.02 Q17.C
  Top 0.305: Q18.1 79.3,27.95
N$30
  Top 0.254: IC3.4 76.97,13.43 | 76.97,13.43 77.5,12.9 77.5,12.12 C3.2 | 76.97,13.43 77.02,13.43 77.5,13.9 77.5,14.65 78.75,15.9 78.75,17.52 79,17.77 80.5,17.77 80.88,17.4 80.88,16.8 R30.2
  Top 0.305: C3.2 77.4,12.25 77.38,12.28 77.38,12.03 C3.2 | C3.2 77.5,12.03
N$31
  Top 0.305: 101.47,33.15 Q19.B | Q20.2 99.4,26.4
  Top 0.406: 99.4,26.4 100.15,27.15 100.15,32.55 R37.1
  Top 0.813: R37.1 101.47,33.15
N$32
  Top 0.254: HP_LED4.4 99.64,19.64 100.4,20.4 100.4,22.9 99.77,23.52 98.02,23.52 97.4,24.15 Q20.3
N$33
  Top 0.254: Q22.3 99.65,15.65 100.02,16.02 100.02,17.52 HP_LED4.5
N$34
  Top 0.305: HP_LED4.6 103.4,18.5 103.4,18.9 103.4,19.4 101.4,21.4 101.4,23.4 101.4,24.9 103.4,26.9 103.4,28.52 Q24.3
N$35  (1 unrouted)
  Top 0.254: 103.9,30.9 104.9,29.9 104.9,27.4 105.4,26.9 106.27,26.9 107.02,26.15 110.4,22.77 110.77,22.77
  Top 0.305: 99.85,24.45 Q20.1 99.95,24.45 102.4,26.9 102.4,29.4 103.9,30.9 103.9,32.17 Q19.C
N$36
  Top 0.254: Q22.2 98.45,16.6 97.65,17.4 97.65,19.45 Q21.B 97.35,19.85 97.65,20.15 97.65,21.25 R40.1
N$37
  Top 0.254: Q22.1 98.02,13.7 R44.2 97.55,13.25 96.15,14.65 96.15,17.3 Q21.C 96.4,17.52 96.15,17.15
N$38
  Top 0.254: Q24.2 106.35,29.85 108.77,32.27 | 108.77,32.27 108.77,32.88 R41.1 | Q23.B 112.35,33.1 111.4,32.15 108.9,32.15 108.77,32.27
N$39
  Top 0.254: Q24.1 105.9,27.9 106.15,27.77 110.15,23.77 111.77,23.77 112.15,23.4 R45.2 | 106.2,27.95 106.2,28.7 108.52,31.02 111.38,31.02 Q23.C
  Top 0.305: Q24.1 106.2,27.95
N$40
  Top 0.254: IC4.4 103.88,13.43 | 103.88,13.43 104.4,12.9 104.4,12.12 C4.2 | 103.88,13.43 103.92,13.43 104.4,13.9 104.4,14.65 105.65,15.9 105.65,17.52 105.9,17.77 107.4,17.77 107.77,17.4 107.77,16.8 R42.2
  Top 0.305: C4.2 104.3,12.25 104.27,12.28 104.27,12.03 C4.2 | C4.2 104.4,12.03
N$41
  Top 0.305: 20.77,67.05 Q25.B | Q26.2 18.7,60.3
  Top 0.406: 18.7,60.3 19.45,61.05 19.45,66.45 R49.1
  Top 0.813: R49.1 20.77,67.05
N$42
  Top 0.254: HP_LED5.4 18.94,53.54 19.7,54.3 19.7,56.8 19.07,57.42 17.32,57.42 16.7,58.05 Q26.3
N$43
  Top 0.254: Q28.3 18.95,49.55 19.32,49.92 19.32,51.42 HP_LED5.5
N$44
  Top 0.305: HP_LED5.6 22.7,52.4 22.7,52.8 22.7,53.3 20.7,55.3 20.7,57.3 20.7,58.8 22.7,60.8 22.7,62.42 Q30.3
N$45  (1 unrouted)
  Top 0.254: 23.2,64.8 24.2,63.8 24.2,61.3 24.7,60.8 25.57,60.8 26.32,60.05 29.7,56.67 30.07,56.67
  Top 0.305: 19.15,58.35 Q26.1 19.25,58.35 21.7,60.8 21.7,63.3 23.2,64.8 23.2,66.08 Q25.C
N$46
  Top 0.254: Q28.2 17.75,50.5 16.95,51.3 16.95,53.35 Q27.B 16.65,53.75 16.95,54.05 16.95,55.15 R52.1
N$47
  Top 0.254: Q28.1 17.32,47.6 R56.2 16.85,47.15 15.45,48.55 15.45,51.2 Q27.C 15.7,51.42 15.45,51.05
N$48
  Top 0.254: Q30.2 25.65,63.75 28.07,66.17 | 28.07,66.17 28.07,66.78 R53.1 | Q29.B 31.65,67 30.7,66.05 28.2,66.05 28.07,66.17
N$49
  Top 0.254: Q30.1 25.2,61.8 25.45,61.67 29.45,57.67 31.07,57.67 31.45,57.3 R57.2 | 25.5,61.85 25.5,62.6 27.82,64.92 30.68,64.92 Q29.C
  Top 0.305: Q30.1 25.5,61.85
N$50
  Top 0.254: IC5.4 23.18,47.33 | 23.18,47.33 23.7,46.8 23.7,46.02 C5.2 | 23.18,47.33 23.23,47.33 23.7,47.8 23.7,48.55 24.95,49.8 24.95,51.42 25.2,51.67 26.7,51.67 27.07,51.3 27.07,50.7 R54.2
  Top 0.305: C5.2 23.6,46.15 23.57,46.17 23.57,45.92 C5.2 | C5.2 23.7,45.92
N$51
  Top 0.305: 47.67,67.05 Q31.B | Q32.2 45.6,60.3
  Top 0.406: 45.6,60.3 46.35,61.05 46.35,66.45 R61.1
  Top 0.813: R61.1 47.67,67.05
N$52
  Top 0.254: HP_LED6.4 45.84,53.54 46.6,54.3 46.6,56.8 45.97,57.42 44.22,57.42 43.6,58.05 Q32.3
N$53
  Top 0.254: Q34.3 45.85,49.55 46.22,49.92 46.22,51.42 HP_LED6.5
N$54
  Top 0.305: HP_LED6.6 49.6,52.4 49.6,52.8 49.6,53.3 47.6,55.3 47.6,57.3 47.6,58.8 49.6,60.8 49.6,62.42 Q36.3
N$55  (1 unrouted)
  Top 0.254: 50.1,64.8 51.1,63.8 51.1,61.3 51.6,60.8 52.47,60.8 53.22,60.05 56.6,56.67 56.97,56.67
  Top 0.305: 46.05,58.35 Q32.1 46.15,58.35 48.6,60.8 48.6,63.3 50.1,64.8 50.1,66.08 Q31.C
N$56
  Top 0.254: Q34.2 44.65,50.5 43.85,51.3 43.85,53.35 Q33.B 43.55,53.75 43.85,54.05 43.85,55.15 R64.1
N$57
  Top 0.254: Q34.1 44.22,47.6 R68.2 43.75,47.15 42.35,48.55 42.35,51.2 Q33.C 42.6,51.42 42.35,51.05
N$58
  Top 0.254: Q36.2 52.55,63.75 54.97,66.17 | 54.97,66.17 54.97,66.78 R65.1 | Q35.B 58.55,67 57.6,66.05 55.1,66.05 54.97,66.17
N$59
  Top 0.254: Q36.1 52.1,61.8 52.35,61.67 56.35,57.67 57.97,57.67 58.35,57.3 R69.2 | 52.4,61.85 52.4,62.6 54.72,64.92 57.57,64.92 Q35.C
  Top 0.305: Q36.1 52.4,61.85
N$60
  Top 0.254: IC6.4 50.07,47.33 | 50.07,47.33 50.6,46.8 50.6,46.02 C6.2 | 50.07,47.33 50.12,47.33 50.6,47.8 50.6,48.55 51.85,49.8 51.85,51.42 52.1,51.67 53.6,51.67 53.97,51.3 53.97,50.7 R66.2
  Top 0.305: C6.2 50.5,46.15 50.47,46.17 50.47,45.92 C6.2 | C6.2 50.6,45.92
N$61
  Top 0.305: 74.58,67.05 Q37.B | Q38.2 72.5,60.3
  Top 0.406: 72.5,60.3 73.25,61.05 73.25,66.45 R73.1
  Top 0.813: R73.1 74.58,67.05
N$62
  Top 0.254: HP_LED7.4 72.74,53.54 73.5,54.3 73.5,56.8 72.88,57.42 71.12,57.42 70.5,58.05 Q38.3
N$63
  Top 0.254: Q40.3 72.75,49.55 73.12,49.92 73.12,51.42 HP_LED7.5
N$64
  Top 0.305: HP_LED7.6 76.5,52.4 76.5,52.8 76.5,53.3 74.5,55.3 74.5,57.3 74.5,58.8 76.5,60.8 76.5,62.42 Q42.3
N$65  (1 unrouted)
  Top 0.254: 77,64.8 78,63.8 78,61.3 78.5,60.8 79.38,60.8 80.12,60.05 83.5,56.67 83.88,56.67
  Top 0.305: 72.95,58.35 Q38.1 73.05,58.35 75.5,60.8 75.5,63.3 77,64.8 77,66.08 Q37.C
N$66
  Top 0.254: Q40.2 71.55,50.5 70.75,51.3 70.75,53.35 Q39.B 70.45,53.75 70.75,54.05 70.75,55.15 R76.1
N$67
  Top 0.254: Q40.1 71.12,47.6 R80.2 70.65,47.15 69.25,48.55 69.25,51.2 Q39.C 69.5,51.42 69.25,51.05
N$68
  Top 0.254: Q42.2 79.45,63.75 81.88,66.17 | 81.88,66.17 81.88,66.78 R77.1 | Q41.B 85.45,67 84.5,66.05 82,66.05 81.88,66.17
N$69
  Top 0.254: Q42.1 79,61.8 79.25,61.67 83.25,57.67 84.88,57.67 85.25,57.3 R81.2 | 79.3,61.85 79.3,62.6 81.62,64.92 84.47,64.92 Q41.C
  Top 0.305: Q42.1 79.3,61.85
N$70
  Top 0.254: IC7.4 76.97,47.33 | 76.97,47.33 77.5,46.8 77.5,46.02 C7.2 | 76.97,47.33 77.02,47.33 77.5,47.8 77.5,48.55 78.75,49.8 78.75,51.42 79,51.67 80.5,51.67 80.88,51.3 80.88,50.7 R78.2
  Top 0.305: C7.2 77.4,46.15 77.38,46.17 77.38,45.92 C7.2 | C7.2 77.5,45.92
N$71
  Top 0.305: 101.47,67.05 Q43.B | Q44.2 99.4,60.3
  Top 0.406: 99.4,60.3 100.15,61.05 100.15,66.45 R85.1
  Top 0.813: R85.1 101.47,67.05
N$72
  Top 0.254: HP_LED8.4 99.64,53.54 100.4,54.3 100.4,56.8 99.77,57.42 98.02,57.42 97.4,58.05 Q44.3
N$73
  Top 0.254: Q46.3 99.65,49.55 100.02,49.92 100.02,51.42 HP_LED8.5
N$74
  Top 0.305: HP_LED8.6 103.4,52.4 103.4,52.8 103.4,53.3 101.4,55.3 101.4,57.3 101.4,58.8 103.4,60.8 103.4,62.42 Q48.3
N$75  (1 unrouted)
  Top 0.254: 103.9,64.8 104.9,63.8 104.9,61.3 105.4,60.8 106.27,60.8 107.02,60.05 110.4,56.67 110.77,56.67
  Top 0.305: 99.85,58.35 Q44.1 99.95,58.35 102.4,60.8 102.4,63.3 103.9,64.8 103.9,66.08 Q43.C
N$76
  Top 0.254: Q46.2 98.45,50.5 97.65,51.3 97.65,53.35 Q45.B 97.35,53.75 97.65,54.05 97.65,55.15 R88.1
N$77
  Top 0.254: Q46.1 98.02,47.6 R92.2 97.55,47.15 96.15,48.55 96.15,51.2 Q45.C 96.4,51.42 96.15,51.05
N$78
  Top 0.254: Q48.2 106.35,63.75 108.77,66.17 | 108.77,66.17 108.77,66.78 R89.1 | Q47.B 112.35,67 111.4,66.05 108.9,66.05 108.77,66.17
N$79
  Top 0.254: Q48.1 105.9,61.8 106.15,61.67 110.15,57.67 111.77,57.67 112.15,57.3 R93.2 | 106.2,61.85 106.2,62.6 108.52,64.92 111.38,64.92 Q47.C
  Top 0.305: Q48.1 106.2,61.85
N$80
  Top 0.254: IC8.4 103.88,47.33 | 103.88,47.33 104.4,46.8 104.4,46.02 C8.2 | 103.88,47.33 103.92,47.33 104.4,47.8 104.4,48.55 105.65,49.8 105.65,51.42 105.9,51.67 107.4,51.67 107.77,51.3 107.77,50.7 R90.2
  Top 0.305: C8.2 104.3,46.15 104.27,46.17 104.27,45.92 C8.2 | C8.2 104.4,45.92
R
  Top 0.254: R3.1 29.68,21.02 28.7,21.02 27.68,20 26.7,19.02 24.7,19.02 24.45,18.77 24.32,18.65 21.95,16.27 IC1.1 21.18,15.38 20.32,14.53 20.32,13.65 19.95,13.28 18.98,13.28 R10.1
R1
  Top 0.254: R19.1 56.57,21.02 55.6,21.02 54.57,20 53.6,19.02 51.6,19.02 51.35,18.77 51.22,18.65 48.85,16.27 IC2.1 48.07,15.38 47.22,14.53 47.22,13.65 46.85,13.28 45.88,13.28 R22.1
R2
  Top 0.254: R31.1 83.47,21.02 82.5,21.02 81.47,20 80.5,19.02 78.5,19.02 78.25,18.77 78.12,18.65 75.75,16.27 IC3.1 74.97,15.38 74.12,14.53 74.12,13.65 73.75,13.28 72.77,13.28 R34.1
R3
  Top 0.254: R43.1 110.38,21.02 109.4,21.02 108.38,20 107.4,19.02 105.4,19.02 105.15,18.77 105.02,18.65 102.65,16.27 IC4.1 101.88,15.38 101.02,14.53 101.02,13.65 100.65,13.28 99.67,13.28 R46.1
R4
  Top 0.254: R55.1 29.68,54.92 28.7,54.92 27.68,53.9 26.7,52.92 24.7,52.92 24.45,52.67 24.32,52.55 21.95,50.17 IC5.1 21.18,49.27 20.32,48.42 20.32,47.55 19.95,47.17 18.98,47.17 R58.1
R5
  Top 0.254: R67.1 56.57,54.92 55.6,54.92 54.57,53.9 53.6,52.92 51.6,52.92 51.35,52.67 51.22,52.55 48.85,50.17 IC6.1 48.07,49.27 47.22,48.42 47.22,47.55 46.85,47.17 45.88,47.17 R70.1
R6
  Top 0.254: R79.1 83.47,54.92 82.5,54.92 81.47,53.9 80.5,52.92 78.5,52.92 78.25,52.67 78.12,52.55 75.75,50.17 IC7.1 74.97,49.27 74.12,48.42 74.12,47.55 73.75,47.17 72.77,47.17 R82.1
R7
  Top 0.254: R91.1 110.38,54.92 109.4,54.92 108.38,53.9 107.4,52.92 105.4,52.92 105.15,52.67 105.02,52.55 102.65,50.17 IC8.1 101.88,49.27 101.02,48.42 101.02,47.55 100.65,47.17 99.67,47.17 R94.1
VCC
  Top 0.254: Q5.E 29.75,33.73 29.45,33.9 26.68,33.9 R5.2 24.68,33.52 22.7,33.52 22.2,33.02 22.2,32.4 21.12,31.32 Q1.E | 25.18,11.9 C1.1 | 25.18,11.9 25.18,14.88 25.7,15.4 | 25.7,15.4 26.07,15.4 | 26.07,15.4 26.43,15.4 IC1.8 | 25.18,11.9 25.18,11.38 24.7,10.9 23.2,10.9 21.7,9.4 | 25.7,15.4 26.07,15.4 | 26.07,15.4 26.07,16.5 R12.2
  pour Top (isolate 0.61, rank 2, no thermals): 23.7,38.9 23.7,6.9 12.2,6.9 12.2,38.9
VCC1
  Top 0.254: Q11.E 56.65,33.73 56.35,33.9 53.57,33.9 R17.2 51.57,33.52 49.6,33.52 49.1,33.02 49.1,32.4 48.02,31.32 Q7.E | 52.07,11.9 C2.1 | 52.07,11.9 52.07,14.88 52.6,15.4 | 52.6,15.4 52.97,15.4 | 52.97,15.4 53.32,15.4 IC2.8 | 52.07,11.9 52.07,11.38 51.6,10.9 50.1,10.9 48.6,9.4 | 52.6,15.4 52.97,15.4 | 52.97,15.4 52.97,16.5 R24.2
  pour Top (isolate 0.61, rank 2, no thermals): 50.6,38.9 50.6,6.9 39.1,6.9 39.1,38.9
VCC2
  Top 0.254: Q17.E 83.55,33.73 83.25,33.9 80.47,33.9 R29.2 78.47,33.52 76.5,33.52 76,33.02 76,32.4 74.92,31.32 Q13.E | 78.97,11.9 C3.1 | 78.97,11.9 78.97,14.88 79.5,15.4 | 79.5,15.4 79.88,15.4 | 79.88,15.4 80.22,15.4 IC3.8 | 78.97,11.9 78.97,11.38 78.5,10.9 77,10.9 75.5,9.4 | 79.5,15.4 79.88,15.4 | 79.88,15.4 79.88,16.5 R36.2
  pour Top (isolate 0.61, rank 2, no thermals): 77.5,38.9 77.5,6.9 66,6.9 66,38.9
VCC3
  Top 0.254: Q23.E 110.45,33.73 110.15,33.9 107.38,33.9 R41.2 105.38,33.52 103.4,33.52 102.9,33.02 102.9,32.4 101.83,31.32 Q19.E | 105.88,11.9 C4.1 | 105.88,11.9 105.88,14.88 106.4,15.4 | 106.4,15.4 106.77,15.4 | 106.77,15.4 107.12,15.4 IC4.8 | 105.88,11.9 105.88,11.38 105.4,10.9 103.9,10.9 102.4,9.4 | 106.4,15.4 106.77,15.4 | 106.77,15.4 106.77,16.5 R48.2
  pour Top (isolate 0.61, rank 2, no thermals): 104.4,38.9 104.4,6.9 92.9,6.9 92.9,38.9
VCC8
  Top 0.254: Q29.E 29.75,67.62 29.45,67.8 26.68,67.8 R53.2 24.68,67.42 22.7,67.42 22.2,66.92 22.2,66.3 21.12,65.22 Q25.E | 25.18,45.8 C5.1 | 25.18,45.8 25.18,48.77 25.7,49.3 | 25.7,49.3 26.07,49.3 | 26.07,49.3 26.43,49.3 IC5.8 | 25.18,45.8 25.18,45.27 24.7,44.8 23.2,44.8 21.7,43.3 | 25.7,49.3 26.07,49.3 | 26.07,49.3 26.07,50.4 R60.2
  pour Top (isolate 0.61, rank 2, no thermals): 23.7,72.8 23.7,40.8 12.2,40.8 12.2,72.8
VCC9
  Top 0.254: Q35.E 56.65,67.62 56.35,67.8 53.57,67.8 R65.2 51.57,67.42 49.6,67.42 49.1,66.92 49.1,66.3 48.02,65.22 Q31.E | 52.07,45.8 C6.1 | 52.07,45.8 52.07,48.77 52.6,49.3 | 52.6,49.3 52.97,49.3 | 52.97,49.3 53.32,49.3 IC6.8 | 52.07,45.8 52.07,45.27 51.6,44.8 50.1,44.8 48.6,43.3 | 52.6,49.3 52.97,49.3 | 52.97,49.3 52.97,50.4 R72.2
  pour Top (isolate 0.61, rank 2, no thermals): 50.6,72.8 50.6,40.8 39.1,40.8 39.1,72.8
VCC10
  Top 0.254: Q41.E 83.55,67.62 83.25,67.8 80.47,67.8 R77.2 78.47,67.42 76.5,67.42 76,66.92 76,66.3 74.92,65.22 Q37.E | 78.97,45.8 C7.1 | 78.97,45.8 78.97,48.77 79.5,49.3 | 79.5,49.3 79.88,49.3 | 79.88,49.3 80.22,49.3 IC7.8 | 78.97,45.8 78.97,45.27 78.5,44.8 77,44.8 75.5,43.3 | 79.5,49.3 79.88,49.3 | 79.88,49.3 79.88,50.4 R84.2
  pour Top (isolate 0.61, rank 2, no thermals): 77.5,72.8 77.5,40.8 66,40.8 66,72.8
VCC11
  Top 0.254: Q47.E 110.45,67.62 110.15,67.8 107.38,67.8 R89.2 105.38,67.42 103.4,67.42 102.9,66.92 102.9,66.3 101.83,65.22 Q43.E | 105.88,45.8 C8.1 | 105.88,45.8 105.88,48.77 106.4,49.3 | 106.4,49.3 106.77,49.3 | 106.77,49.3 107.12,49.3 IC8.8 | 105.88,45.8 105.88,45.27 105.4,44.8 103.9,44.8 102.4,43.3 | 106.4,49.3 106.77,49.3 | 106.77,49.3 106.77,50.4 R96.2
  pour Top (isolate 0.61, rank 2, no thermals): 104.4,72.8 104.4,40.8 92.9,40.8 92.9,72.8
(copper drawn outside any net)
  shapes: Top circle x16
